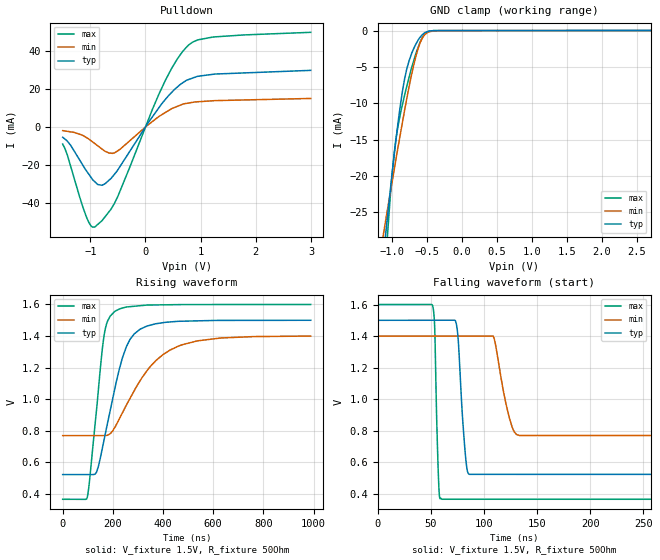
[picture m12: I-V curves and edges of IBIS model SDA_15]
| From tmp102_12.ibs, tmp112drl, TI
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|   SDA_15  1.8V digital I/O open drain Model
[Model] SDA_15
Model_type   I/O_open_drain
| Signals   SDA(6)
Polarity   Non-Inverting
Enable   Active-Low
Vinl = 0.45
Vinh = 1.05
Vmeas = 0.75
Vref = 0.75
Cref = 15pF
Rref = 50
|   typ   min   max
|   (nom PVT)   (Fast PVT)   (slow PVT)
|   output low
|C_comp   1.5414960e-10  7.6379100e-11  2.5474710e-10
| Where   nom PVT is  Nominal Process, 1.5V, 27C
|   Fast PVT is Strong Process, 1.6V, 125C
|   Slow PVT is Weak Process, 1.4V, -40C
|   output high
C_comp   1.4373800e-12  1.4323490e-12  1.4406010e-12
| Where   nom PVT is  Nominal Process, 1.5V, 27C
|   Fast PVT is Strong Process, 1.6V, -40C
|   Slow PVT is Weak Process, 1.4V, 125C
[Voltage Range]   1.5   1.4   1.6
[Temperature Range]   27   125   -40
|Ambient Temperature   27   125   -40
[Pullup Reference]   1.5   1.4   1.6
[Pulldown Reference]   0   0   0
[Power Clamp Reference]   1.5   1.4   1.6
[GND Clamp Reference]   0   0   0
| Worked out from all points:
|   slope of the pulldown table from 0 to 0.225 V, typ, clamps not added: 24 ohm
|   GND clamp passes 1 mA (typ) near -0.60 V on its own axis
|   falling waveform, V_fixture 1.5V, R_fixture 50Ohm: 20-80 % time 5.21ns typ, 10.7ns min, 2.6ns max; typ from 1.5 V to 0.522 V
|   rising waveform, V_fixture 1.5V, R_fixture 50Ohm: 20-80 % time 85.7ns typ, 161ns min, 45.7ns max; typ from 0.522 V to 1.5 V
[Pulldown]
|   Voltage   I(typ)   I(min)   I(max)
-1.5V     -5.376mA   -1.887mA   -8.965mA
-1.415V   -7.468mA   -2.273mA   -14.74mA
-1.072V   -22.86mA   -5.492mA   -46.95mA
-989.9mV  -26.24mA   -7.114mA   -51.73mA
-918mV    -28.7mA    -8.687mA   -52.39mA
-785.9mV  -30.51mA   -11.58mA   -49mA
-557.3mV  -24.6mA    -13.52mA   -39.74mA
243.5mV   10.08mA    5.496mA    17.18mA
471.9mV   18.03mA    9.567mA    30.58mA
772.7mV   24.79mA    12.52mA    42.72mA
1.225V    27.62mA    13.76mA    47.16mA
2.995V    29.68mA    14.96mA    49.62mA
[GND Clamp]
|   Voltage   I(typ)   I(min)   I(max)
-1.5V     -68.31mA   -50.89mA   -99.84mA
-1.107V   -29.85mA   -27.31mA   -34.82mA
-1.081V   -27.43mA   -25.76mA   -31mA
-1.056V   -25.11mA   -24.32mA   -27.42mA
-1.011V   -21.06mA   -21.74mA   -21.56mA
-963.6mV  -16.97mA   -19.03mA   -16.71mA
-910.2mV  -12.65mA   -16.03mA   -13.1mA
-816mV    -6.621mA   -10.91mA   -8.868mA
-754.4mV  -4.204mA   -7.831mA   -6.505mA
-650.1mV  -1.78mA    -3.353mA   -3.006mA
-524.5mV  -273.7uA   -532.6uA   -472.9uA
2.995V    0A         0A         0A
[POWER Clamp]
|   SCR cell for ESD function. Effects occurr above VDD x 2
|   Voltage   I(typ)   I(min)   I(max)
-1.5V     0A         0A         0A
0V        0A         0A         0A
3V        0A         0A         0A
[Ramp]
R_load = 50
|   typ   min   max
dV/dt_r   0.586721/8.51973e-008  0.378665/1.60627e-007  0.740874/4.55683e-008
dV/dt_f   0.586721/5.1976e-009   0.378665/1.06843e-008  0.740874/2.58987e-009
[Falling Waveform]
V_fixture = 1.5V
V_fixture_min = 1.4V
V_fixture_max = 1.6V
R_fixture = 50Ohm
C_fixture = 0F
|   Time   V(typ)   V(min)   V(max)
0s        1.5V       1.4V       1.6V
51.61ns   1.5V       1.4V       1.594V
53.6ns    1.5V       1.4V       1.449V
57.5ns    1.5V       1.4V       443.5mV
60.47ns   1.5V       1.4V       365.7mV
73.84ns   1.482V     1.4V       365.7mV
86.28ns   523.7mV    1.4V       365.7mV
109.4ns   523.6mV    1.389V     365.7mV
133.3ns   523.6mV    770.1mV    365.7mV
988.6ns   522.1mV    768.9mV    365.2mV
[Rising Waveform]
V_fixture = 1.5V
V_fixture_min = 1.4V
V_fixture_max = 1.6V
R_fixture = 50Ohm
C_fixture = 0F
|   Time   V(typ)   V(min)   V(max)
0s        522.1mV    768.9mV    365.2mV
97.71ns   522.1mV    768.9mV    376.3mV
134ns     534.5mV    768.9mV    917.2mV
163.7ns   732.6mV    768.9mV    1.39V
178.8ns   848.7mV    771.4mV    1.495V
205.5ns   1.049V     815.2mV    1.553V
267.6ns   1.376V     1.003V     1.586V
335.1ns   1.463V     1.178V     1.596V
536.7ns   1.496V     1.369V     1.6V
988.6ns   1.5V       1.4V       1.6V
